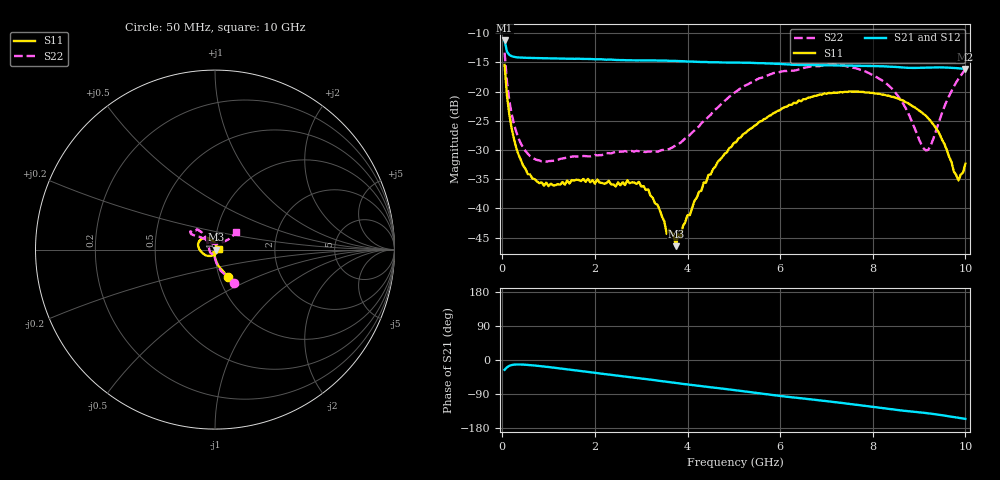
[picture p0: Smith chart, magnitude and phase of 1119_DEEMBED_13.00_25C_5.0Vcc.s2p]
!Hittite Microwave Corp.
!Digital Attenuator/PhaseShifter Rev 1.4.0
!Filename: C:\DATA\DATA\1119_DEEMBED_13.00_25C_5.0Vcc.s2p
!VNA ID: Agilent Technologies,N5224A,MY51441122,A.10.45.03
!Device type:
!2 Port Calibration.
!Temp(C): 25
!Lot Number:
!Serial Number:
!Operator:
!Misc:
!Attenuator:  13.000
# GHZ S DB R 50.0
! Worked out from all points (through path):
!   200 points, 50 MHz to 10 GHz, reference 50 ohm
!   highest |S21| = -11.25 dB at 50 MHz (marker M1); lowest = -16.1 dB at 10 GHz (marker M2)
!   group delay of S21, straight-line fit = 41.1 ps
!   lowest |S11| = -46.5 dB at 3.75 GHz (marker M3), VSWR 1.01, Z = 50.5 - j0.0634 ohm
!   |S11| at or under -10 dB: start of sweep to end of sweep
!   |S22| runs from -32.0 to -13.3 dB; largest |S21 - S12| = 0.00063
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0.05  -15.43 -64.4  -11.25 -25.8  -11.25 -25.8  -13.33 -59.8
0.1  -20.60 -78.1  -13.15 -19.4  -13.15 -19.4  -18.24 -74.8
0.2  -26.23 -88.1  -13.93 -13.4  -13.93 -13.4  -23.73 -86.1
0.35  -30.79 -94.8  -14.16 -11.8  -14.15 -11.8  -27.98 -92.8
0.55  -34.11 -102.5  -14.23 -12.9  -14.23 -12.9  -30.63 -98.8
1  -36.17 -111.7  -14.31 -18.6  -14.31 -18.6  -31.90 -106.7
1.75  -34.95 -116.5  -14.41 -29.8  -14.41 -29.9  -31.02 -115.0
2.95  -35.45 -92.9  -14.65 -47.9  -14.66 -48.0  -30.20 -152.3
3.4  -40.27 -78.6  -14.69 -55.0  -14.69 -55.0  -30.14 -174.6
3.55  -44.34 -53.8  -14.70 -57.6  -14.71 -57.6  -29.93 176.9
3.7  -44.55 -28.9  -14.74 -59.8  -14.75 -59.9  -29.43 168.6
3.75  -46.45 -7.6  -14.76 -60.7  -14.77 -60.7  -29.21 166.1
3.8  -44.33 -4.1  -14.77 -61.5  -14.78 -61.5  -28.98 162.3
4.35  -35.56 59.2  -14.93 -69.6  -14.94 -69.7  -25.05 137.4
5.05  -28.64 92.2  -15.04 -80.0  -15.06 -80.0  -19.99 126.6
6.7  -20.85 135.5  -15.46 -104.3  -15.47 -104.3  -15.66 139.7
7.65  -19.98 158.4  -15.58 -118.2  -15.59 -118.2  -16.03 146.9
8.35  -20.71 173.2  -15.73 -129.0  -15.73 -129.0  -19.01 140.6
9.15  -24.12 -150.2  -15.90 -139.9  -15.91 -139.9  -30.08 90.0
9.45  -27.41 -123.4  -15.85 -144.9  -15.87 -144.9  -24.72 44.2
9.85  -35.19 -36.2  -16.01 -152.5  -16.02 -152.5  -17.83 38.1
10  -32.33 11.9  -16.12 -155.4  -16.13 -155.4  -16.21 39.3
